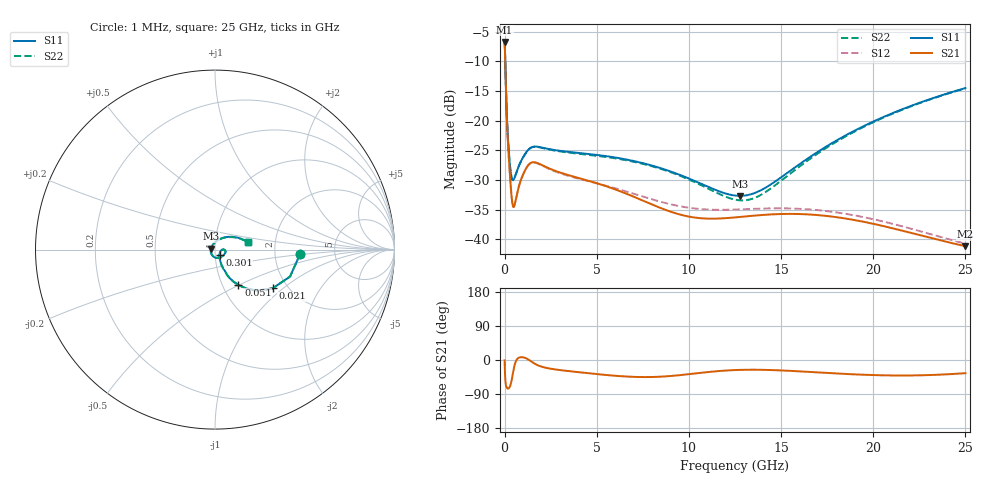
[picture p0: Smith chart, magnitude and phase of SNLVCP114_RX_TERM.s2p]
! Touchstone Ver. 1.0
! Mon Jun 18 17:48:36 2012
! Number of ports is 2
# Hz	S	MA	R	50.000000
! SCATTERING PARAMETERS  :
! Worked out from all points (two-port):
!   2501 points, 1 MHz to 25 GHz, reference 50 ohm
!   highest |S21| = -6.72 dB at 1 MHz (marker M1); lowest = -41.2 dB at 25 GHz (marker M2)
!   |S21| within 3 dB of the highest: start of sweep to 29.31 MHz
!   lowest |S11| = -32.7 dB at 12.79 GHz (marker M3), VSWR 1.05, Z = 47.8 + j0.517 ohm
!   |S11| at or under -10 dB: 33 MHz to end of sweep
!   |S22| runs from -33.5 to -6.5 dB; largest |S21 - S12| = 0.0031
!   S11 on the Smith chart (normalised r, x): 1 MHz: 2.80, -0.17; 21 MHz: 1.67, -0.85; 51 MHz: 1.19, -0.50; 301 MHz: 1.05, -0.07; 25 GHz: 1.44, +0.13
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1000000  0.475 -2.8  0.4612 -1.0  0.4612 -1.0  0.475 -2.8
2.1e7  0.3866 -34.0  0.3754 -35.0  0.3754 -35.0  0.3866 -34.0
5.1e7  0.2364 -56.5  0.2291 -59.2  0.2291 -59.2  0.2364 -56.5
1.41e8  0.09329 -67.0  0.08847 -74.6  0.08848 -74.6  0.09329 -67.0
1.81e8  0.07125 -65.5  0.06629 -75.6  0.06628 -75.7  0.07124 -65.5
2.41e8  0.05153 -60.0  0.04562 -74.0  0.0456 -74.0  0.05151 -60.1
3.01e8  0.04031 -51.3  0.03276 -68.5  0.03273 -68.6  0.04027 -51.4
4.11e8  0.03198 -30.8  0.02064 -46.6  0.02058 -46.6  0.03193 -30.8
5.11e8  0.03222 -14.9  0.01887 -20.3  0.0188 -20.1  0.03216 -14.8
1.001e9  0.04896 0.3  0.03506 7.1  0.03498 7.4  0.04886 0.5
1.241e9  0.05574 -3.8  0.04125 2.6  0.04113 3.0  0.0556 -3.5
1.471e9  0.05966 -10.4  0.04432 -4.8  0.04415 -4.4  0.05947 -10.1
4.171e9  0.05308 -51.1  0.0323 -32.9  0.03193 -30.0  0.05225 -49.6
8.341e9  0.04027 -102.7  0.01864 -44.3  0.02093 -38.5  0.03976 -98.6
1.0331e10  0.03089 -133.2  0.0152 -35.5  0.01812 -33.9  0.03019 -128.1
1.2501e10  0.02333 175.3  0.01525 -26.5  0.01776 -29.5  0.02155 179.7
1.2791e10  0.02318 166.5  0.01539 -26.1  0.01783 -29.3  0.02125 170.3
1.4021e10  0.02643 129.8  0.01601 -25.9  0.01811 -30.0  0.02419 130.5
1.6671e10  0.05056 78.9  0.0161 -31.8  0.01775 -36.4  0.04883 77.8
1.8631e10  0.07694 57.6  0.01481 -37.1  0.01623 -42.1  0.07554 56.7
2.0841e10  0.1121 39.6  0.01257 -40.7  0.01372 -46.8  0.1109 39.0
2.5001e10  0.1882 13.0  0.008721 -34.8  0.009145 -44.0  0.1874 12.7
